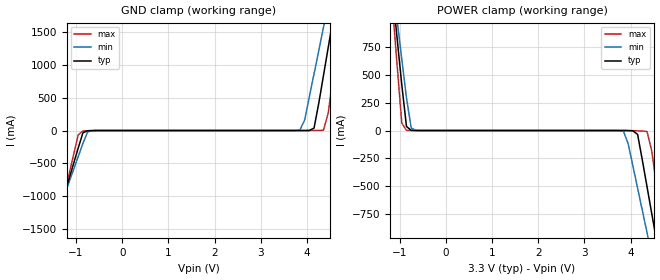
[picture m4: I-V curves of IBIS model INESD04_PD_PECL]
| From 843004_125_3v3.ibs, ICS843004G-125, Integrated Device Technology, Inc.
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[Model]   INESD04_PD_PECL
Model_type   Input
Polarity   Non-Inverting
Vinl = 0.8V
Vinh = 2V
|   typ   min   max
C_comp   2pF   1.5pF   2.5pF
|   typ   min   max
[Voltage range]  3.3V   3.135V   3.465V
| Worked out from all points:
|   GND clamp passes 1 mA (typ) near -0.66 V on its own axis
|   POWER clamp passes 1 mA (typ) near -0.73 V on its own axis
[GND_clamp]
|Voltage   I(typ)   I(min)   I(max)
-3.3V     -5.814A    -5.014A    -7.153A
-1.565V   -1.712A    -1.599A    -1.915A
-1.463V   -1.471A    -1.398A    -1.607A
-952.6mV  -265.5mA   -395.3mA   -65.86mA
-850.5mV  -35.06mA   -195.2mA   -6.413mA
-646.4mV  -767.5uA   -1.073mA   -1.657mA
3.844V    85.86uA    6.63mA     58.07uA
4.151V    36.56mA    861.2mA    220uA
4.355V    835.1mA    1.564A     4.863mA
4.559V    1.68A      2.268A     803.2mA
4.763V    2.526A     2.972A     1.885A
6.6V      10.15A     9.315A     11.63A
[POWER_clamp]
|Voltage   I(typ)   I(min)   I(max)
-3.3V     10.15A     8.745A     12.5A
-1.157V   1.258A     1.347A     1.137A
-1.055V   835.1mA    995.9mA    596.1mA
-952.6mV  412.8mA    644.6mA    67.23mA
-850.5mV  36.56mA    293.4mA    1.923mA
-646.4mV  176.2uA    988.6uA    133uA
3.844V    -172uA     -6.351mA   -13.6uA
4.151V    -35.06mA   -518.7mA   -2.36mA
4.355V    -506.4mA   -919.6mA   -9.532mA
4.559V    -988.6mA   -1.321A    -492mA
4.763V    -1.471A    -1.722A    -1.108A
6.6V      -5.814A    -5.339A    -6.655A
